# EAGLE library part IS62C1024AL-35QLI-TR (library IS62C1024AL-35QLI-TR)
SRAM 1Mb 128K x 8 35ns 5v Async SRAM 5v Source: Datasheet
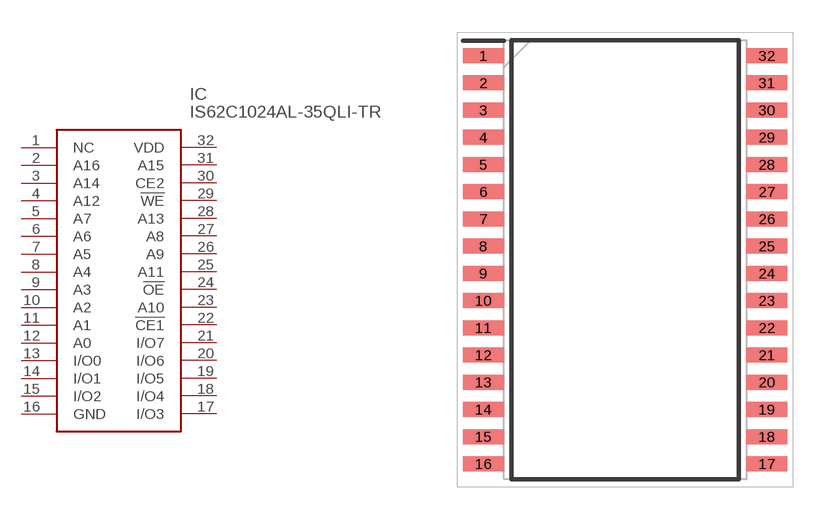
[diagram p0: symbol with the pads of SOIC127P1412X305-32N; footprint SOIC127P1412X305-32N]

Designator prefix IC

## IS62C1024AL-35QLI-TR (Description: SRAM 1Mb 128K x 8 35ns 5v Async SRAM 5v; Height: 3.05mm; Manufacturer_Name: Integrated Silicon Solution Inc.; Manufacturer_Part_Number: IS62C1024AL-35QLI-TR; Mouser_Part_Number: 870IS62C1024AL35QLIT; Mouser_Price-Stock: https://www.mouser.co.uk/ProductDetail/ISSI/IS62C1024AL-35QLI-TR?qs=tFgq3%2FJV4HgOUVNChCblDw%3D%3D)  [SOIC127P1412X305-32N]
1  NC  nc
2  A16
3  A14
4  A12
5  A7
6  A6
7  A5
8  A4
9  A3
10  A2
11  A1
12  A0
13  I/O0
14  I/O1
15  I/O2
16  GND
17  I/O3
18  I/O4
19  I/O5
20  I/O6
21  I/O7
22  !CE1
23  A10
24  !OE
25  A11
26  A9
27  A8
28  A13
29  !WE
30  CE2
31  A15
32  VDD

## Footprint SOIC127P1412X305-32N (pad centres in mm)
32L 450MIL SOP REV.F
smd 1.922 x 0.7: 1 -6.614,9.525; 2 -6.614,8.255; 3 -6.614,6.985; 4 -6.614,5.715; 5 -6.614,4.445; 6 -6.614,3.175; 7 -6.614,1.905; 8 -6.614,0.635; 9 -6.614,-0.635; 10 -6.614,-1.905; 11 -6.614,-3.175; 12 -6.614,-4.445; 13 -6.614,-5.715; 14 -6.614,-6.985; 15 -6.614,-8.255; 16 -6.614,-9.525; 17 6.614,-9.525; 18 6.614,-8.255; 19 6.614,-6.985; 20 6.614,-5.715; 21 6.614,-4.445; 22 6.614,-3.175; 23 6.614,-1.905; 24 6.614,-0.635; 25 6.614,0.635; 26 6.614,1.905; 27 6.614,3.175; 28 6.614,4.445; 29 6.614,5.715; 30 6.614,6.985; 31 6.614,8.255; 32 6.614,9.525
